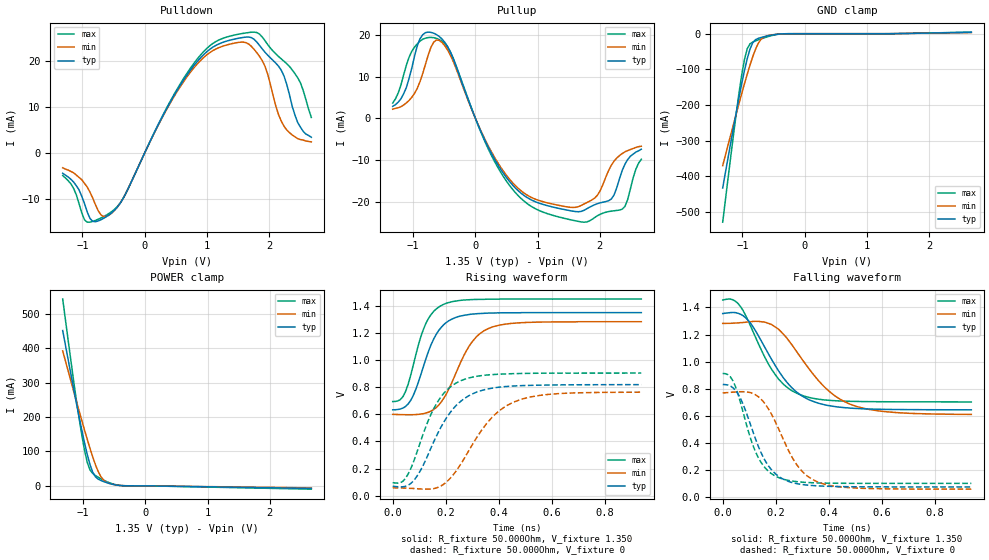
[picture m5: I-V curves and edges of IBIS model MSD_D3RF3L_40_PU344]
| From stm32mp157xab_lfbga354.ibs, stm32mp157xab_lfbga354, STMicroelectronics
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[Model] MSD_D3RF3L_40_PU344
Model_type   I/O
C_comp 2.337pF   2.253pF   2.460pF
Vinh = 810.000mV
Vinl = 540.000mV
Vmeas = 675.000mV
Vref = 675.000mV
[Model Spec]
Vinh   810.000mV   777.000mV   860.000mV
Vinl   540.000mV   507.000mV   590.000mV
Vmeas   675.000mV   642.000mV   725.000mV
Vref   675.000mV   642.000mV   725.000mV
[Temperature Range]   25.000   125.000   -40.000
[Voltage Range]   1.350V   1.283V   1.450V
[GND Clamp Reference]   0.00V   0.00V   0.00V
[Pulldown Reference]   0.00V   0.00V   0.00V
[POWER Clamp Reference]   1.350V   1.283V   1.450V
[Pullup Reference]   1.350V   1.283V   1.450V
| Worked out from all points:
|   slope of the pulldown table from 0 to 0.203 V, typ, clamps not added: 35.6 ohm
|   slope of the pullup table from 0 to 0.203 V, typ, clamps not added: 29.7 ohm
|   GND clamp passes 1 mA (typ) near -0.41 V on its own axis
|   POWER clamp passes 1 mA (typ) near -0.41 V on its own axis
|   rising waveform, R_fixture 50.000Ohm, V_fixture 1.350: 20-80 % time 84.1ps typ, 107ps min, 71.1ps max; typ from 0.633 V to 1.35 V
|   rising waveform, R_fixture 50.000Ohm, V_fixture 0: 20-80 % time 128ps typ, 154ps min, 108ps max; typ from 0.069 V to 0.819 V
|   falling waveform, R_fixture 50.000Ohm, V_fixture 1.350: 20-80 % time 144ps typ, 173ps min, 124ps max; typ from 1.35 V to 0.644 V
|   falling waveform, R_fixture 50.000Ohm, V_fixture 0: 20-80 % time 96.2ps typ, 115ps min, 83.1ps max; typ from 0.831 V to 0.075 V
[GND Clamp]
-1.318V   -432.7mA   -370.2mA   -528.8mA
-1.142V   -260.6mA   -252.7mA   -280.1mA
-1.055V   -178.2mA   -195.2mA   -165.1mA
-1.011V   -139mA     -167.2mA   -114.1mA
-966.7mV  -102.3mA   -139.7mA   -71.22mA
-922.7mV  -69.47mA   -113.2mA   -41.62mA
-878.8mV  -42.87mA   -87.88mA   -28.25mA
-834.9mV  -25.29mA   -64.47mA   -23.34mA
-790.9mV  -16.82mA   -43.84mA   -20.18mA
-703mV    -10.74mA   -15.95mA   -14.58mA
-527.3mV  -3.867mA   -3.267mA   -5.173mA
2.68V     3.846mA    3.267mA    4.549mA
[Power Clamp]
-1.33V    452.1mA    392.8mA    543.8mA
-1.155V   283.1mA    276.1mA    306.4mA
-1.023V   162.2mA    190.3mA    147.9mA
-978.8mV  125.1mA    162.4mA    103.4mA
-934.9mV  91.05mA    135.1mA    67.96mA
-890.9mV  61.71mA    108.8mA    46.37mA
-847mV    39.4mA     83.89mA    35.92mA
-759.1mV  19.48mA    41.52mA    24.95mA
-671.2mV  12.28mA    16.32mA    16.36mA
-583.3mV  7.022mA    7.054mA    9.286mA
-451.5mV  1.801mA    2.042mA    2.252mA
2.668V    -7.581mA   -6.072mA   -9.749mA
[Pulldown]
-1.318V   -4.4mA     -3.2mA     -4.9mA
-922.7mV  -12.81mA   -7.4mA     -14.99mA
-703mV    -14.46mA   -13.41mA   -14.07mA
-571.2mV  -13.38mA   -13.45mA   -13.08mA
-351.5mV  -9.978mA   -9.967mA   -9.956mA
747mV     18.14mA    17.69mA    18.58mA
1.098V    22.94mA    22.18mA    23.74mA
1.582V    25.02mA    24.02mA    25.9mA
1.933V    21.85mA    18.84mA    24.36mA
2.241V    16.67mA    5.8mA      19.86mA
2.461V    6.6mA      3.1mA      16.3mA
2.68V     3.4mA      2.4mA      7.7mA
[Pullup]
-1.33V    2.9mA      2.205mA    3.679mA
-1.111V   7.4mA      3.715mA    12.77mA
-978.8mV  15mA       6.025mA    17.13mA
-715.1mV  20.68mA    17.11mA    19.47mA
-451.5mV  17.37mA    16.56mA    17.25mA
251.5mV   -8.25mA    -7.87mA    -8.717mA
866.7mV   -19.34mA   -18.74mA   -20.85mA
1.702V    -22.36mA   -20.93mA   -24.89mA
1.965V    -20.49mA   -18.41mA   -23.38mA
2.185V    -19.39mA   -11.27mA   -22.3mA
2.361V    -12.5mA    -8.438mA   -21.82mA
2.668V    -7.4mA     -6.7mA     -9.821mA
[Ramp]
R_load=50.000Ohm
dV/dt_r   435.081mV/106.000ps  414.456mV/130.500ps  465.240mV/90.000ps
dV/dt_f   435.081mV/121.000ps  414.456mV/145.500ps  465.240mV/104.000ps
[Rising waveform]
R_fixture=50.000Ohm
V_fixture=1.350
V_fixture_min=1.283
V_fixture_max=1.450
0s        633.2mV    599.7mV    694.2mV
39ps      646.3mV    597.3mV    731.2mV
68ps      703.2mV    596.9mV    888.6mV
106ps     891.8mV    602mV      1.172V
125ps     1.008V     609.6mV    1.27V
154ps     1.153V     634.2mV    1.358V
192ps     1.26V      716.7mV    1.411V
288ps     1.336V     1.102V     1.445V
374ps     1.347V     1.243V     1.449V
938ps     1.35V      1.283V     1.45V
[Rising waveform]
R_fixture=50.000Ohm
V_fixture=0
0s        69.19mV    58.16mV    95.66mV
48ps      68.74mV    55.65mV    127.4mV
87ps      130.6mV    51.63mV    295mV
163ps     431.8mV    55.94mV    670.6mV
211ps     597.5mV    116.1mV    791.3mV
259ps     699.6mV    239.2mV    849.7mV
355ps     785.2mV    533.6mV    889.6mV
460ps     809.1mV    692.8mV    900.1mV
614ps     816.6mV    751.1mV    903.6mV
938ps     818.7mV    763.2mV    904.1mV
[Falling waveform]
R_fixture=50.000Ohm
V_fixture=1.350
V_fixture_min=1.283
V_fixture_max=1.450
0s        1.355V     1.282V     1.455V
48ps      1.362V     1.285V     1.446V
96ps      1.305V     1.293V     1.302V
192ps     991.3mV    1.264V     921.7mV
240ps     853.1mV    1.179V     814.7mV
288ps     761.9mV    1.049V     759.2mV
393ps     677.6mV    796mV      715.7mV
489ps     655.8mV    679.7mV    706.7mV
652ps     646.5mV    624.2mV    703.4mV
938ps     644.3mV    610mV      702.4mV
[Falling waveform]
R_fixture=50.000Ohm
V_fixture=0
0s        830.8mV    768.8mV    912.3mV
29ps      820.1mV    773.1mV    887.6mV
48ps      788.4mV    776mV      816.6mV
77ps      684.8mV    777.9mV    625.9mV
125ps     422.5mV    753.6mV    329mV
163ps     258.7mV    679.3mV    209.4mV
202ps     166.7mV    541.3mV    151.7mV
288ps     96.16mV    216.3mV    112.1mV
374ps     81.12mV    100.5mV    103.6mV
938ps     74.84mV    58.29mV    101.1mV
